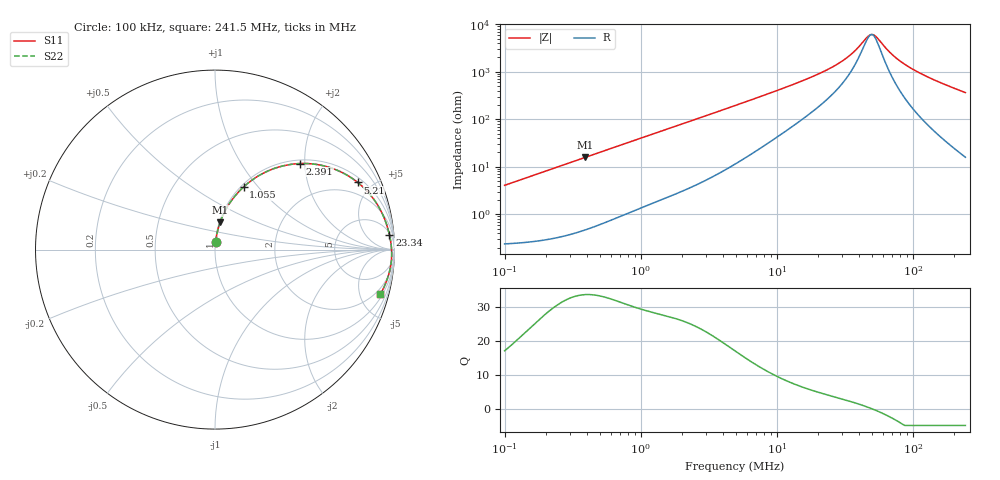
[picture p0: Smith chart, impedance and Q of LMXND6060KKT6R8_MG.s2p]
! LMXND6060KKT6R8_MG  S-PARAMETER MODEL  ( General Type )
! Model Generated by TAIYO YUDEN Corporation (https://www.yuden.co.jp/en/)
! Version 1.0
! TAIYO YUDEN Control No. 191023NI43SB-FBB
! Copyright(c) 2019 TAIYO YUDEN CO.,LTD. All Rights Reserved.
! Product Description (link to TY-COMPAS)
! https://ds.yuden.co.jp/TYCOMPAS/or/detail?pn=LMXND6060KKT6R8MMG&u=M
! Products Name : Inductors
! Characteristics :
!  Inductance : 6.8 uH , SRF(min) : 30 MHz , DC Resistance(max) : 0.264 Ohm
!  Rated Current : Saturation :1200 mA , Temp Rise : 1200 mA (40 degC)
!  Case Size : 6.0 x 6.0 / 0.236 x 0.236 [mm/inch] , Thickness : 1 / 0.039 [mm/inch]
!  (Conditions: Temperature = 25 degC , DC Bias Current/Voltage = 0A / 0V)
! External Node Assignments :
!  1  o---GGG---o  2
! GND o---------o GND
! Frequency Range : 0.1MHz  -  241.513628MHz  [ 402 STEP ]
# MHz S RI R 50
! Freq[MHz].  S11 Real  S11 Imag  S21 Real  S21 Imag  S12 Real  S12 Imag  S22 Real  S22 Imag
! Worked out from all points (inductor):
!   401 points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, 100 kHz to 241.5 MHz, reference 50 ohm
!   read as one part in series: L = 6.47 uH near 104 kHz
!   highest Q = 33.7 at 390.9 kHz (marker M1), where L = 6.44 uH
!   self-resonance near 49.3 MHz
!   S11 on the Smith chart (normalised r, x): 100 kHz: 1.00, +0.08; 1.055 MHz: 1.03, +0.84; 2.391 MHz: 1.08, +1.89; 5.21 MHz: 1.25, +4.11; 23.34 MHz: 6, +21; 241.5 MHz: 1.32, -7.28
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0.1  0.00401 0.0404  0.996 -0.0404  0.996 -0.0404  0.00401 0.0404
0.368674  0.0259 0.1448  0.9741 -0.1448  0.9741 -0.1448  0.0259 0.1448
0.390854  0.0287 0.1529  0.9713 -0.1529  0.9713 -0.1529  0.0287 0.1529
0.67425  0.0753 0.2487  0.9247 -0.2487  0.9247 -0.2487  0.0753 0.2487
1.055212  0.1592 0.3491  0.8408 -0.3491  0.8408 -0.3491  0.1592 0.3491
1.359207  0.2341 0.4059  0.7659 -0.4059  0.7659 -0.4059  0.2341 0.4059
2.39083  0.4724 0.4795  0.5276 -0.4795  0.5276 -0.4795  0.4724 0.4795
3.329076  0.6272 0.461  0.3728 -0.461  0.3728 -0.461  0.6272 0.461
4.914404  0.7771 0.3879  0.2229 -0.3879  0.2229 -0.3879  0.7771 0.3879
5.210062  0.7951 0.3743  0.2049 -0.3743  0.2049 -0.3743  0.7951 0.3743
8.987705  0.9084 0.2446  0.0916 -0.2446  0.0916 -0.2446  0.9084 0.2446
18.11814  0.9629 0.1177  0.0371 -0.1177  0.0371 -0.1177  0.9629 0.1177
23.33776  0.9715 0.0838  0.0285 -0.0838  0.0285 -0.0838  0.9715 0.0838
33.13535  0.9792 0.043  0.0208 -0.043  0.0208 -0.043  0.9792 0.043
46.13883  0.9834 0.00719  0.0166 -0.00719  0.0166 -0.00719  0.9834 0.00719
48.91461  0.9838 0.000863  0.0162 -0.000863  0.0162 -0.000863  0.9838 0.000863
53.91696  0.9843 -0.0098  0.0157 0.0098  0.0157 0.0098  0.9843 -0.0098
66.79689  0.9844 -0.0341  0.0156 0.0341  0.0156 0.0341  0.9844 -0.0341
82.75365  0.9827 -0.0603  0.0173 0.0603  0.0173 0.0603  0.9827 -0.0603
108.6901  0.9775 -0.0978  0.0225 0.0978  0.0225 0.0978  0.9775 -0.0978
157.3547  0.9615 -0.1592  0.0385 0.1592  0.0385 0.1592  0.9615 -0.1592
241.5136  0.9206 -0.2494  0.0794 0.2494  0.0794 0.2494  0.9206 -0.2494
